(* Logix 5000 AddOnInstructionDefinition export Banner_Q90R2_KD_Param_v4; software revision 33.00; part 3 of 3 *)
(* tags used below, declared in another part *)
   Q90R2KD : Banner_Q90R2KD_v4;
   Port_Data : Banner_IOL_Port_v4;
   Port : DINT;
   Local_Control : DINT;
   Command_Being_Processed : BOOL;
   Index_Write_Inprocess : DINT;
   Inprocess_Index : DINT;
(* Banner_Q90R2_KD_Param_v4, continued *)

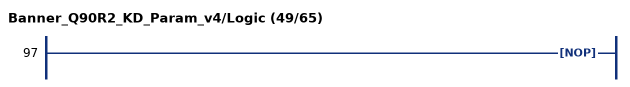
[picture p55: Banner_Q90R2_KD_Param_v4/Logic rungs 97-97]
   97: NOP();
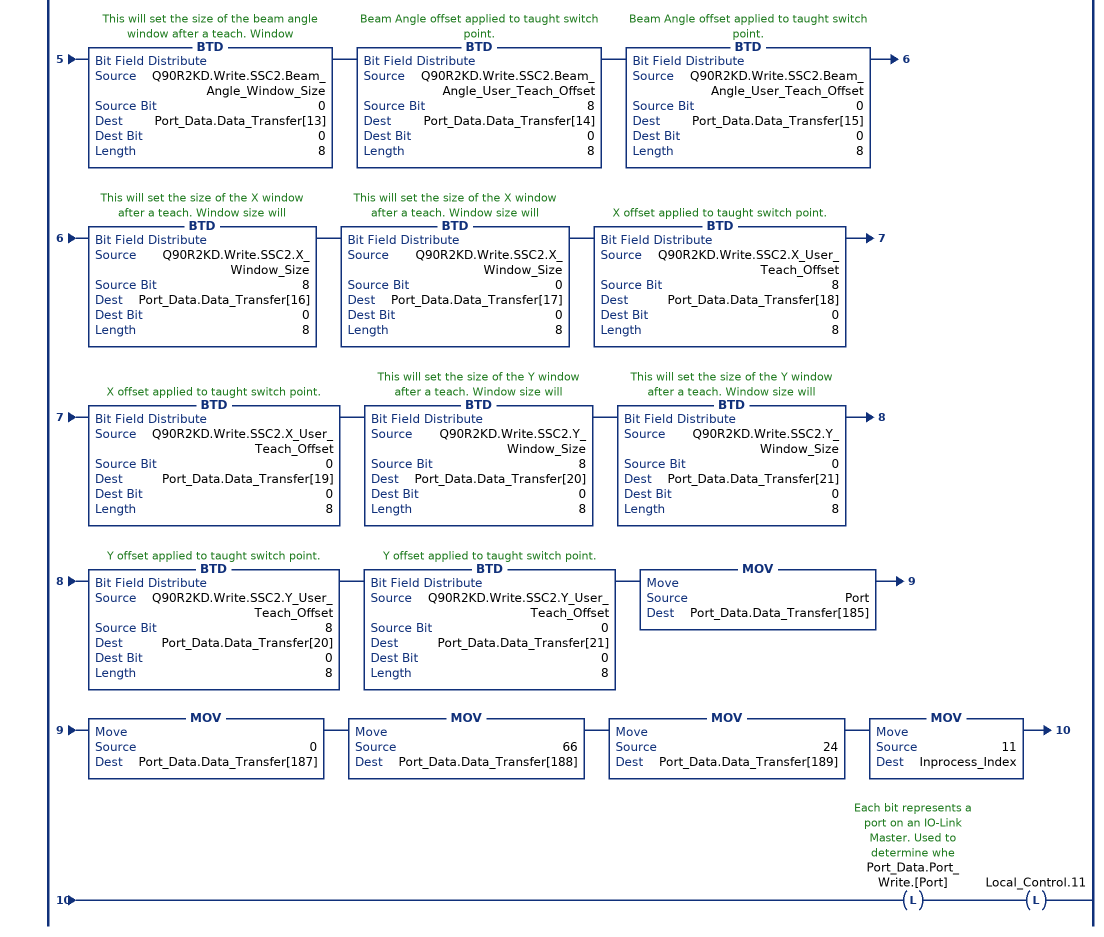
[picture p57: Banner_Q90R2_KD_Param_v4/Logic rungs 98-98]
   // ************************************************************************************************************
   // Section of AOI that controls writing of the SSC2 Vendor Specific Configuration parameter (index 66).
   // ************************************************************************************************************
   98: XIC(Q90R2KD.Initial_Global_Read)XIO(Command_Being_Processed)XIO(Local_Control.11)EQU(Q90R2KD.Command,50)OTL(Command_Being_Processed)BTD(Q90R2KD.Write.SSC2.Delay_On,24,Port_Data.Data_Transfer[0],0,8)BTD(Q90R2KD.Write.SSC2.Delay_On,16,Port_Data.Data_Transfer[1],0,8)BTD(Q90R2KD.Write.SSC2.Delay_On,8,Port_Data.Data_Transfer[2],0,8)BTD(Q90R2KD.Write.SSC2.Delay_On,0,Port_Data.Data_Transfer[3],0,8)BTD(Q90R2KD.Write.SSC2.Delay_Off,24,Port_Data.Data_Transfer[4],0,8)BTD(Q90R2KD.Write.SSC2.Delay_Off,16,Port_Data.Data_Transfer[5],0,8)BTD(Q90R2KD.Write.SSC2.Delay_Off,8,Port_Data.Data_Transfer[6],0,8)BTD(Q90R2KD.Write.SSC2.Delay_Off,0,Port_Data.Data_Transfer[7],0,8)BTD(Q90R2KD.Write.SSC2.Distance_Window_Size,8,Port_Data.Data_Transfer[8],0,8)BTD(Q90R2KD.Write.SSC2.Distance_Window_Size,0,Port_Data.Data_Transfer[9],0,8)BTD(Q90R2KD.Write.SSC2.Distance_User_Teach_Offset,8,Port_Data.Data_Transfer[10],0,8)BTD(Q90R2KD.Write.SSC2.Distance_User_Teach_Offset,0,Port_Data.Data_Transfer[11],0,8)BTD(Q90R2KD.Write.SSC2.Beam_Angle_Window_Size,8,Port_Data.Data_Transfer[12],0,8)BTD(Q90R2KD.Write.SSC2.Beam_Angle_Window_Size,0,Port_Data.Data_Transfer[13],0,8)BTD(Q90R2KD.Write.SSC2.Beam_Angle_User_Teach_Offset,8,Port_Data.Data_Transfer[14],0,8)BTD(Q90R2KD.Write.SSC2.Beam_Angle_User_Teach_Offset,0,Port_Data.Data_Transfer[15],0,8)BTD(Q90R2KD.Write.SSC2.X_Window_Size,8,Port_Data.Data_Transfer[16],0,8)BTD(Q90R2KD.Write.SSC2.X_Window_Size,0,Port_Data.Data_Transfer[17],0,8)BTD(Q90R2KD.Write.SSC2.X_User_Teach_Offset,8,Port_Data.Data_Transfer[18],0,8)BTD(Q90R2KD.Write.SSC2.X_User_Teach_Offset,0,Port_Data.Data_Transfer[19],0,8)BTD(Q90R2KD.Write.SSC2.Y_Window_Size,8,Port_Data.Data_Transfer[20],0,8)BTD(Q90R2KD.Write.SSC2.Y_Window_Size,0,Port_Data.Data_Transfer[21],0,8)BTD(Q90R2KD.Write.SSC2.Y_User_Teach_Offset,8,Port_Data.Data_Transfer[20],0,8)BTD(Q90R2KD.Write.SSC2.Y_User_Teach_Offset,0,Port_Data.Data_Transfer[21],0,8)MOV(Port,Port_Data.Data_Transfer[185])MOV(0,Port_Data.Data_Transfer[187])MOV(66,Port_Data.Data_Transfer[188])MOV(24,Port_Data.Data_Transfer[189])MOV(11,Inprocess_Index)OTL(Port_Data.Port_Write.[Port])OTL(Local_Control.11);
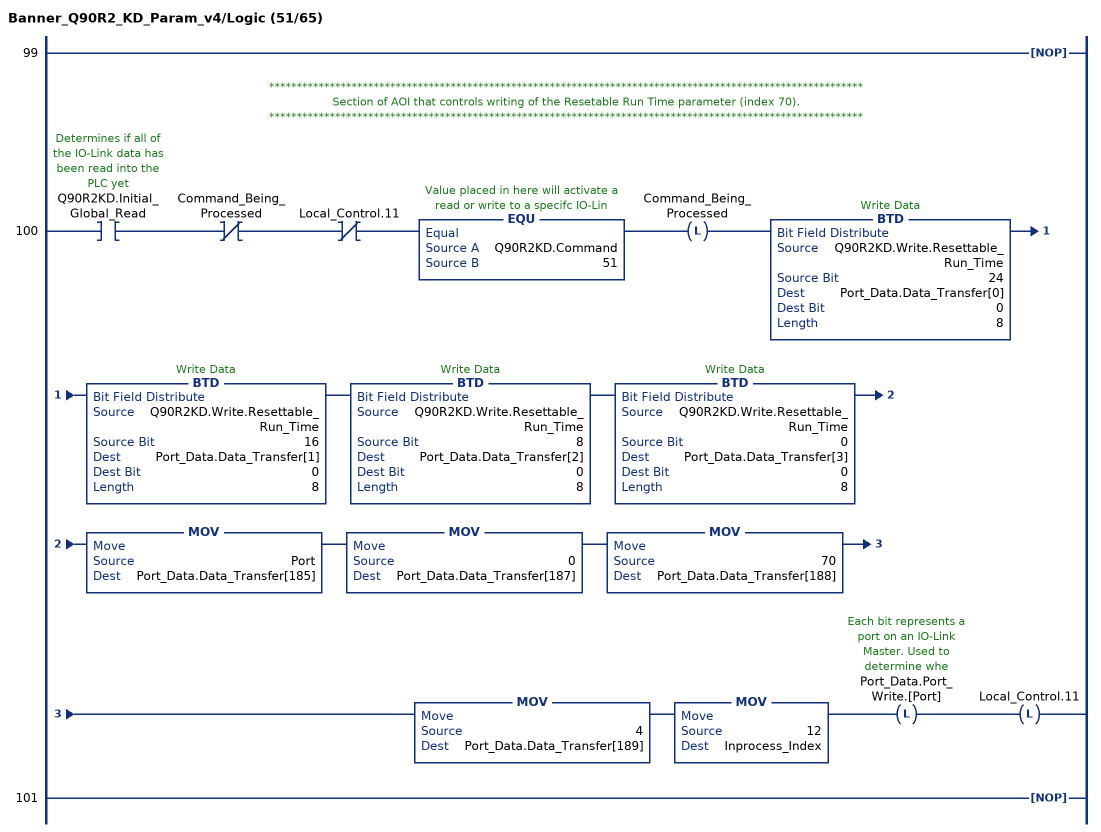
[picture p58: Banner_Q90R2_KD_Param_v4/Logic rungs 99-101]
   99: NOP();
   // ************************************************************************************************************
   // Section of AOI that controls writing of the Resetable Run Time parameter (index 70).
   // ************************************************************************************************************
   100: XIC(Q90R2KD.Initial_Global_Read)XIO(Command_Being_Processed)XIO(Local_Control.11)EQU(Q90R2KD.Command,51)OTL(Command_Being_Processed)BTD(Q90R2KD.Write.Resettable_Run_Time,24,Port_Data.Data_Transfer[0],0,8)BTD(Q90R2KD.Write.Resettable_Run_Time,16,Port_Data.Data_Transfer[1],0,8)BTD(Q90R2KD.Write.Resettable_Run_Time,8,Port_Data.Data_Transfer[2],0,8)BTD(Q90R2KD.Write.Resettable_Run_Time,0,Port_Data.Data_Transfer[3],0,8)MOV(Port,Port_Data.Data_Transfer[185])MOV(0,Port_Data.Data_Transfer[187])MOV(70,Port_Data.Data_Transfer[188])MOV(4,Port_Data.Data_Transfer[189])MOV(12,Inprocess_Index)OTL(Port_Data.Port_Write.[Port])OTL(Local_Control.11);
   101: NOP();
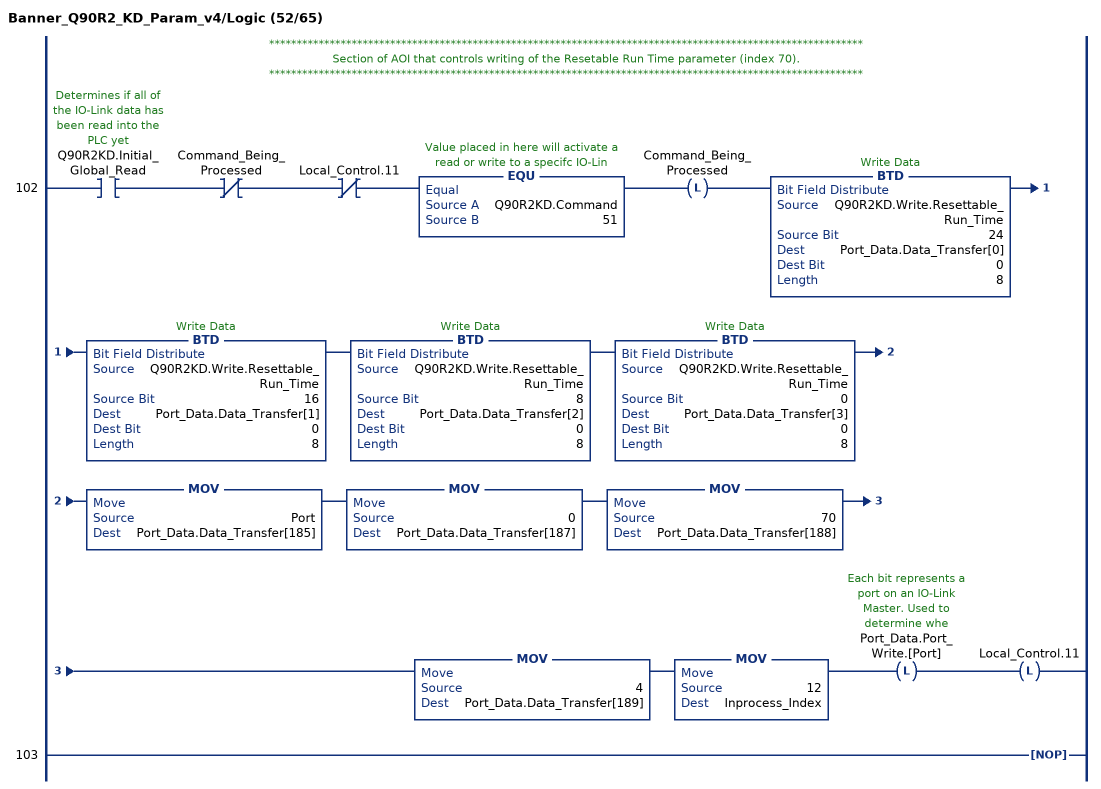
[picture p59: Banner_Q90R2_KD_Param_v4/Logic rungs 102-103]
   // ************************************************************************************************************
   // Section of AOI that controls writing of the Resetable Run Time parameter (index 70).
   // ************************************************************************************************************
   102: XIC(Q90R2KD.Initial_Global_Read)XIO(Command_Being_Processed)XIO(Local_Control.11)EQU(Q90R2KD.Command,51)OTL(Command_Being_Processed)BTD(Q90R2KD.Write.Resettable_Run_Time,24,Port_Data.Data_Transfer[0],0,8)BTD(Q90R2KD.Write.Resettable_Run_Time,16,Port_Data.Data_Transfer[1],0,8)BTD(Q90R2KD.Write.Resettable_Run_Time,8,Port_Data.Data_Transfer[2],0,8)BTD(Q90R2KD.Write.Resettable_Run_Time,0,Port_Data.Data_Transfer[3],0,8)MOV(Port,Port_Data.Data_Transfer[185])MOV(0,Port_Data.Data_Transfer[187])MOV(70,Port_Data.Data_Transfer[188])MOV(4,Port_Data.Data_Transfer[189])MOV(12,Inprocess_Index)OTL(Port_Data.Port_Write.[Port])OTL(Local_Control.11);
   103: NOP();
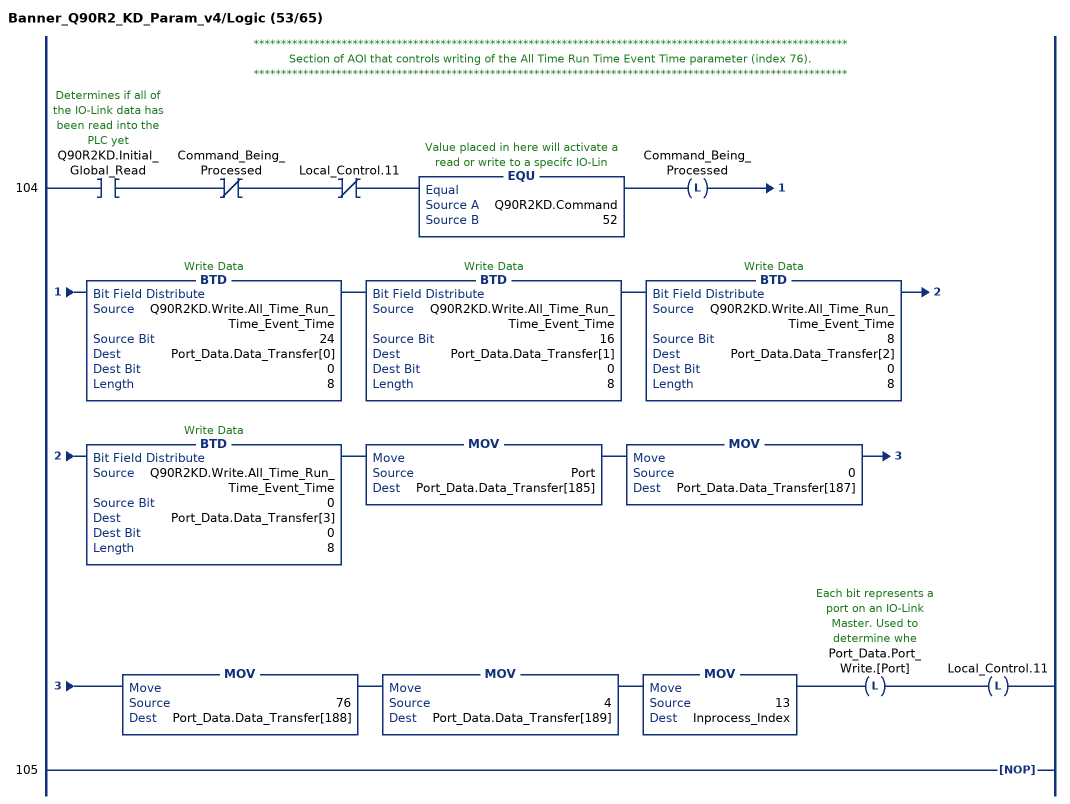
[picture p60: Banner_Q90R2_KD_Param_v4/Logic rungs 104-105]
   // ************************************************************************************************************
   // Section of AOI that controls writing of the All Time Run Time Event Time parameter (index 76).
   // ************************************************************************************************************
   104: XIC(Q90R2KD.Initial_Global_Read)XIO(Command_Being_Processed)XIO(Local_Control.11)EQU(Q90R2KD.Command,52)OTL(Command_Being_Processed)BTD(Q90R2KD.Write.All_Time_Run_Time_Event_Time,24,Port_Data.Data_Transfer[0],0,8)BTD(Q90R2KD.Write.All_Time_Run_Time_Event_Time,16,Port_Data.Data_Transfer[1],0,8)BTD(Q90R2KD.Write.All_Time_Run_Time_Event_Time,8,Port_Data.Data_Transfer[2],0,8)BTD(Q90R2KD.Write.All_Time_Run_Time_Event_Time,0,Port_Data.Data_Transfer[3],0,8)MOV(Port,Port_Data.Data_Transfer[185])MOV(0,Port_Data.Data_Transfer[187])MOV(76,Port_Data.Data_Transfer[188])MOV(4,Port_Data.Data_Transfer[189])MOV(13,Inprocess_Index)OTL(Port_Data.Port_Write.[Port])OTL(Local_Control.11);
   105: NOP();
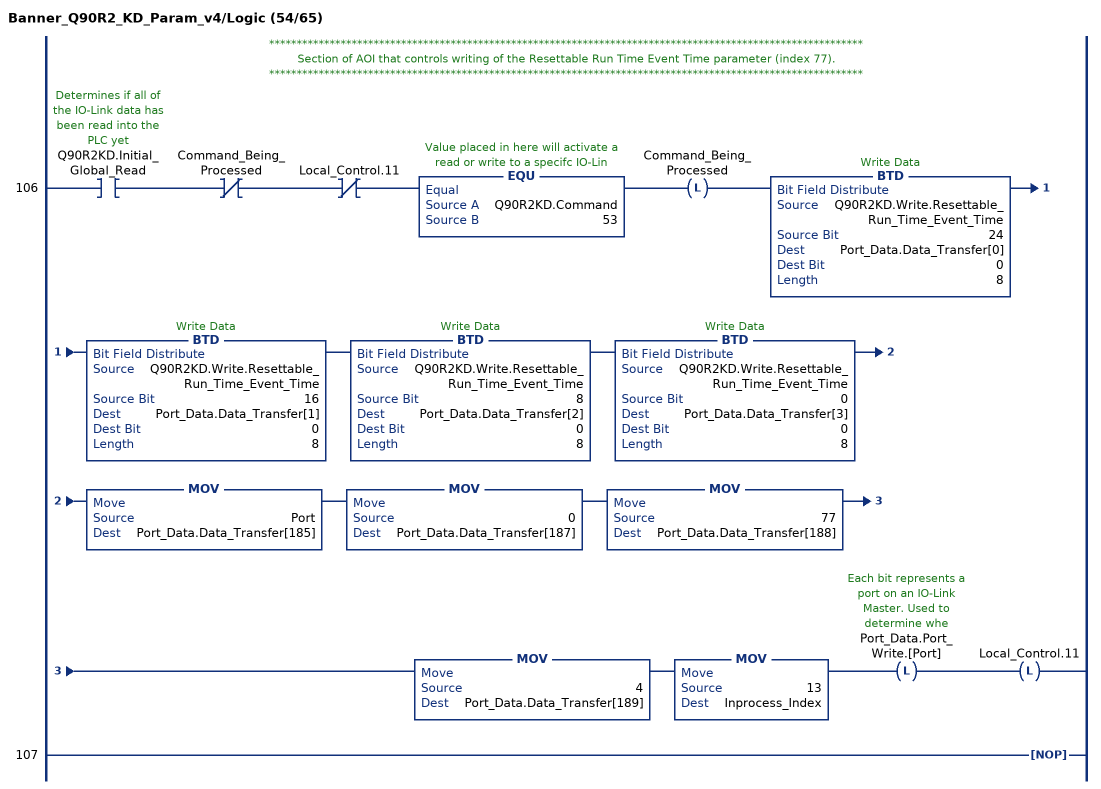
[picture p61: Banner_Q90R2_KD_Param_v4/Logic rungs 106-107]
   // ************************************************************************************************************
   // Section of AOI that controls writing of the Resettable Run Time Event Time parameter (index 77).
   // ************************************************************************************************************
   106: XIC(Q90R2KD.Initial_Global_Read)XIO(Command_Being_Processed)XIO(Local_Control.11)EQU(Q90R2KD.Command,53)OTL(Command_Being_Processed)BTD(Q90R2KD.Write.Resettable_Run_Time_Event_Time,24,Port_Data.Data_Transfer[0],0,8)BTD(Q90R2KD.Write.Resettable_Run_Time_Event_Time,16,Port_Data.Data_Transfer[1],0,8)BTD(Q90R2KD.Write.Resettable_Run_Time_Event_Time,8,Port_Data.Data_Transfer[2],0,8)BTD(Q90R2KD.Write.Resettable_Run_Time_Event_Time,0,Port_Data.Data_Transfer[3],0,8)MOV(Port,Port_Data.Data_Transfer[185])MOV(0,Port_Data.Data_Transfer[187])MOV(77,Port_Data.Data_Transfer[188])MOV(4,Port_Data.Data_Transfer[189])MOV(13,Inprocess_Index)OTL(Port_Data.Port_Write.[Port])OTL(Local_Control.11);
   107: NOP();
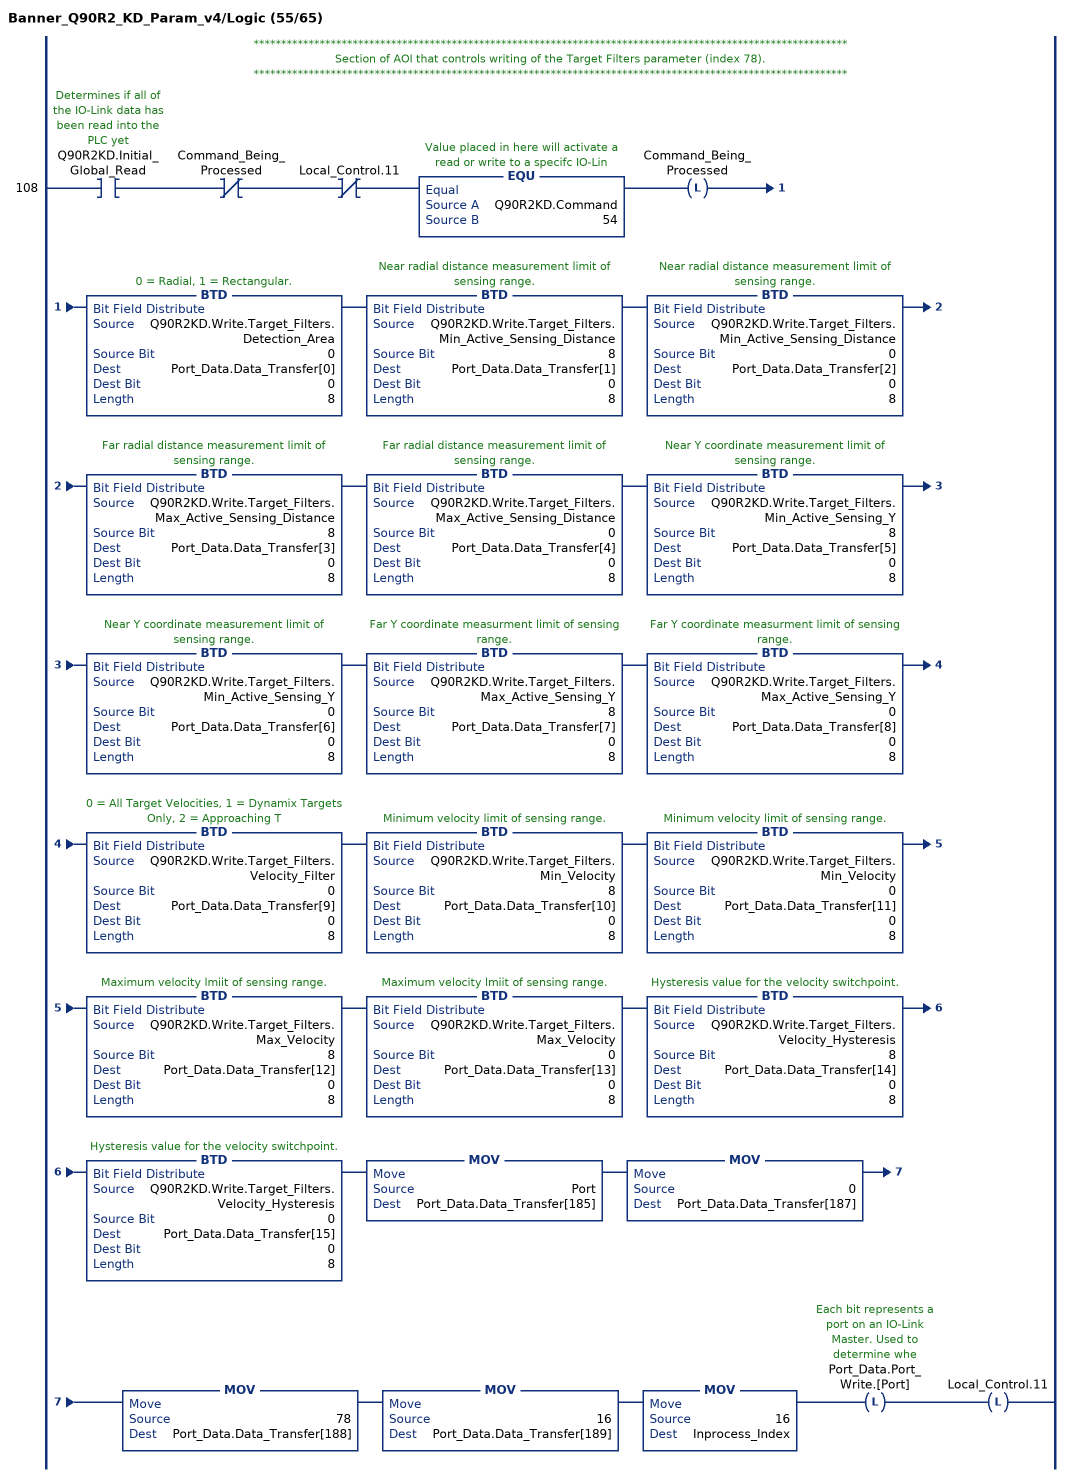
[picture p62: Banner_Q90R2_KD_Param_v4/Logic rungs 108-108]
   // ************************************************************************************************************
   // Section of AOI that controls writing of the Target Filters parameter (index 78).
   // ************************************************************************************************************
   108: XIC(Q90R2KD.Initial_Global_Read)XIO(Command_Being_Processed)XIO(Local_Control.11)EQU(Q90R2KD.Command,54)OTL(Command_Being_Processed)BTD(Q90R2KD.Write.Target_Filters.Detection_Area,0,Port_Data.Data_Transfer[0],0,8)BTD(Q90R2KD.Write.Target_Filters.Min_Active_Sensing_Distance,8,Port_Data.Data_Transfer[1],0,8)BTD(Q90R2KD.Write.Target_Filters.Min_Active_Sensing_Distance,0,Port_Data.Data_Transfer[2],0,8)BTD(Q90R2KD.Write.Target_Filters.Max_Active_Sensing_Distance,8,Port_Data.Data_Transfer[3],0,8)BTD(Q90R2KD.Write.Target_Filters.Max_Active_Sensing_Distance,0,Port_Data.Data_Transfer[4],0,8)BTD(Q90R2KD.Write.Target_Filters.Min_Active_Sensing_Y,8,Port_Data.Data_Transfer[5],0,8)BTD(Q90R2KD.Write.Target_Filters.Min_Active_Sensing_Y,0,Port_Data.Data_Transfer[6],0,8)BTD(Q90R2KD.Write.Target_Filters.Max_Active_Sensing_Y,8,Port_Data.Data_Transfer[7],0,8)BTD(Q90R2KD.Write.Target_Filters.Max_Active_Sensing_Y,0,Port_Data.Data_Transfer[8],0,8)BTD(Q90R2KD.Write.Target_Filters.Velocity_Filter,0,Port_Data.Data_Transfer[9],0,8)BTD(Q90R2KD.Write.Target_Filters.Min_Velocity,8,Port_Data.Data_Transfer[10],0,8)BTD(Q90R2KD.Write.Target_Filters.Min_Velocity,0,Port_Data.Data_Transfer[11],0,8)BTD(Q90R2KD.Write.Target_Filters.Max_Velocity,8,Port_Data.Data_Transfer[12],0,8)BTD(Q90R2KD.Write.Target_Filters.Max_Velocity,0,Port_Data.Data_Transfer[13],0,8)BTD(Q90R2KD.Write.Target_Filters.Velocity_Hysteresis,8,Port_Data.Data_Transfer[14],0,8)BTD(Q90R2KD.Write.Target_Filters.Velocity_Hysteresis,0,Port_Data.Data_Transfer[15],0,8)MOV(Port,Port_Data.Data_Transfer[185])MOV(0,Port_Data.Data_Transfer[187])MOV(78,Port_Data.Data_Transfer[188])MOV(16,Port_Data.Data_Transfer[189])MOV(16,Inprocess_Index)OTL(Port_Data.Port_Write.[Port])OTL(Local_Control.11);
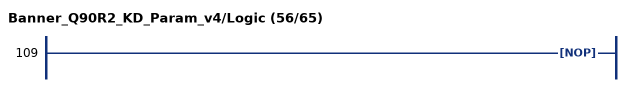
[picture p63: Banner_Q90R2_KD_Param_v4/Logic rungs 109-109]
   109: NOP();
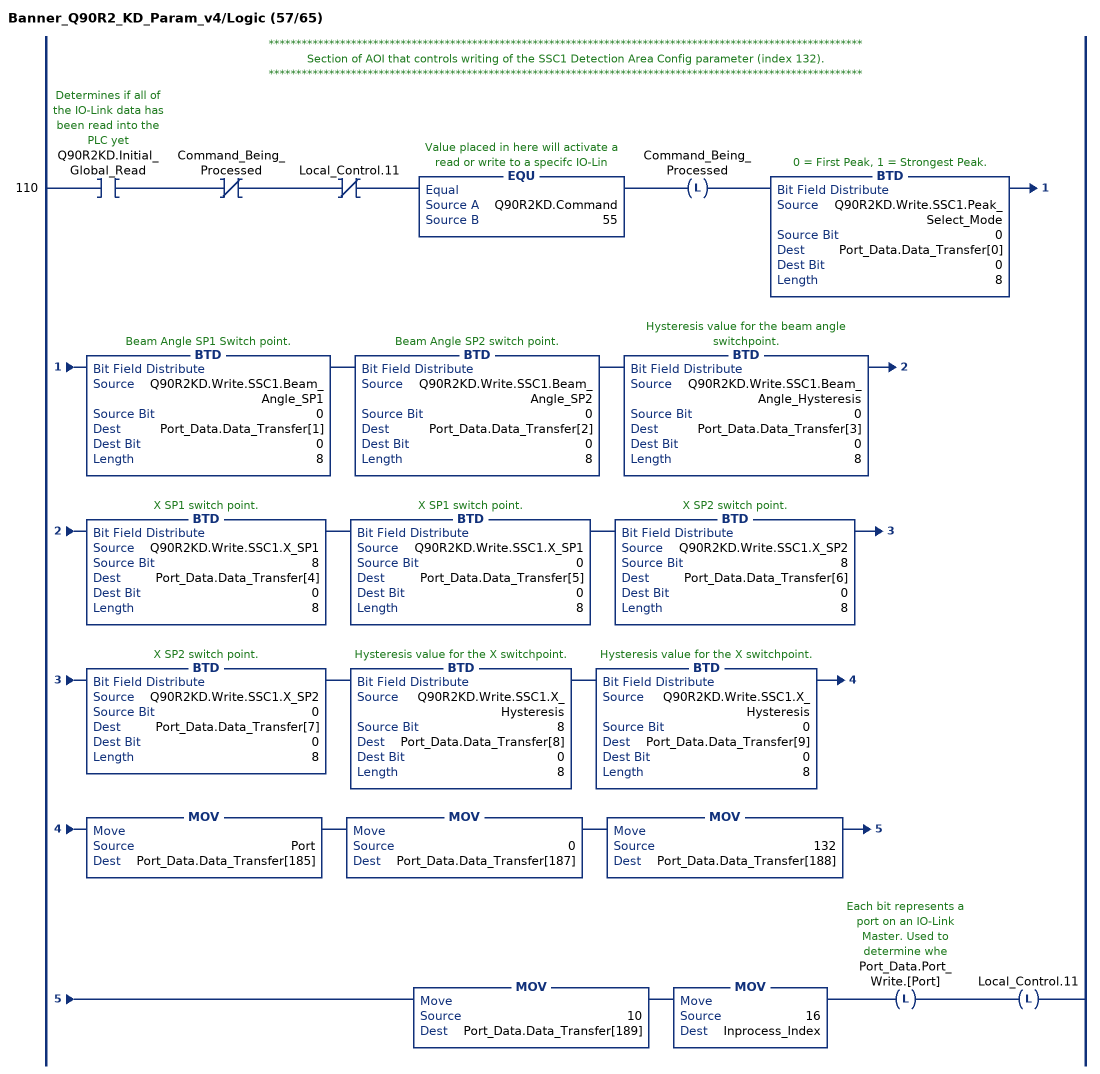
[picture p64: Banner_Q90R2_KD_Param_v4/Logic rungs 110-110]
   // ************************************************************************************************************
   // Section of AOI that controls writing of the SSC1 Detection Area Config parameter (index 132).
   // ************************************************************************************************************
   110: XIC(Q90R2KD.Initial_Global_Read)XIO(Command_Being_Processed)XIO(Local_Control.11)EQU(Q90R2KD.Command,55)OTL(Command_Being_Processed)BTD(Q90R2KD.Write.SSC1.Peak_Select_Mode,0,Port_Data.Data_Transfer[0],0,8)BTD(Q90R2KD.Write.SSC1.Beam_Angle_SP1,0,Port_Data.Data_Transfer[1],0,8)BTD(Q90R2KD.Write.SSC1.Beam_Angle_SP2,0,Port_Data.Data_Transfer[2],0,8)BTD(Q90R2KD.Write.SSC1.Beam_Angle_Hysteresis,0,Port_Data.Data_Transfer[3],0,8)BTD(Q90R2KD.Write.SSC1.X_SP1,8,Port_Data.Data_Transfer[4],0,8)BTD(Q90R2KD.Write.SSC1.X_SP1,0,Port_Data.Data_Transfer[5],0,8)BTD(Q90R2KD.Write.SSC1.X_SP2,8,Port_Data.Data_Transfer[6],0,8)BTD(Q90R2KD.Write.SSC1.X_SP2,0,Port_Data.Data_Transfer[7],0,8)BTD(Q90R2KD.Write.SSC1.X_Hysteresis,8,Port_Data.Data_Transfer[8],0,8)BTD(Q90R2KD.Write.SSC1.X_Hysteresis,0,Port_Data.Data_Transfer[9],0,8)MOV(Port,Port_Data.Data_Transfer[185])MOV(0,Port_Data.Data_Transfer[187])MOV(132,Port_Data.Data_Transfer[188])MOV(10,Port_Data.Data_Transfer[189])MOV(16,Inprocess_Index)OTL(Port_Data.Port_Write.[Port])OTL(Local_Control.11);
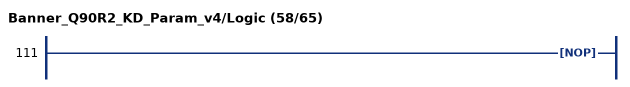
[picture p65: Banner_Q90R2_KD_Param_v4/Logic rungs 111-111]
   111: NOP();
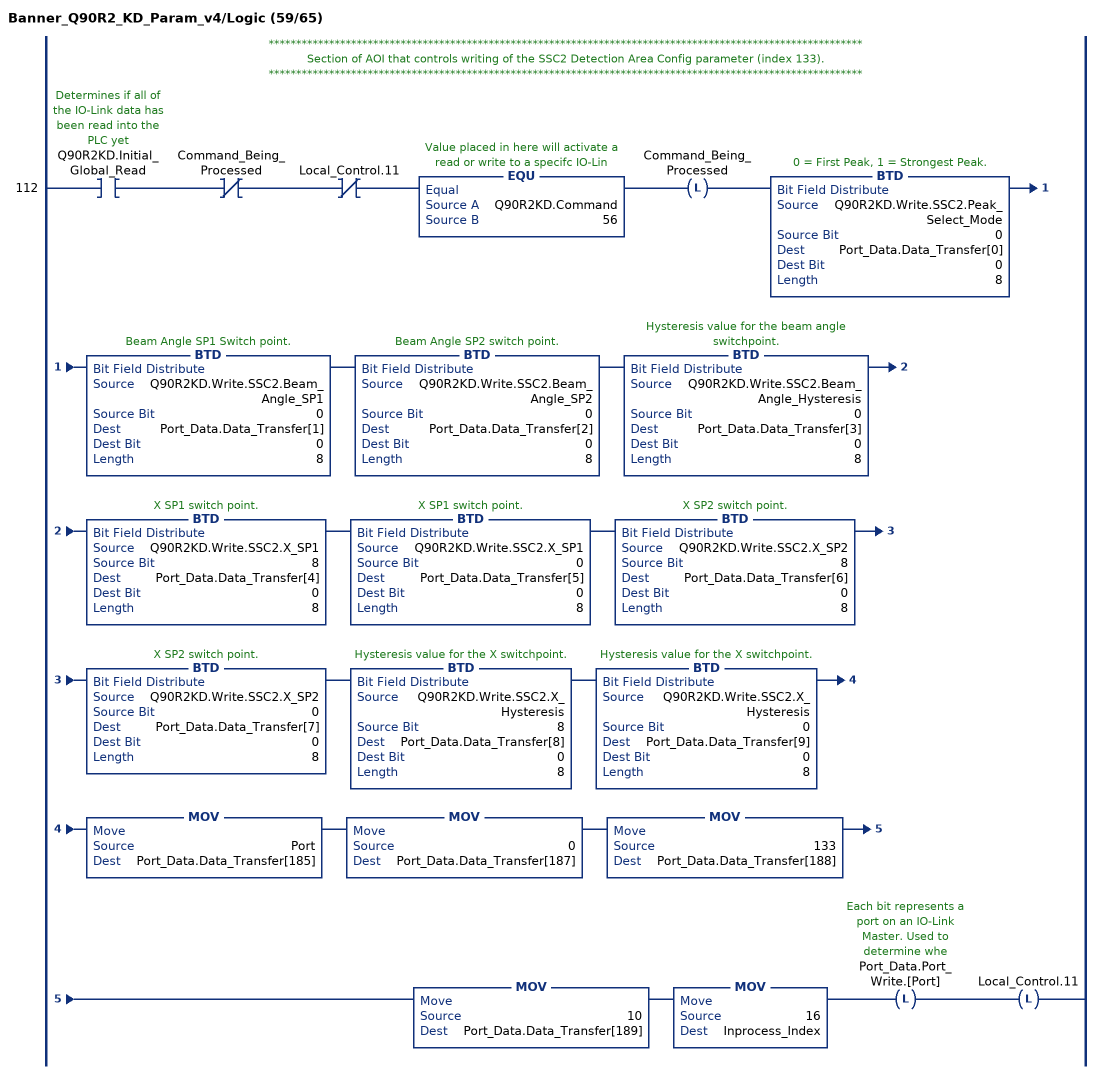
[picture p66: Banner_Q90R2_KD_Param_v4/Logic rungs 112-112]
   // ************************************************************************************************************
   // Section of AOI that controls writing of the SSC2 Detection Area Config parameter (index 133).
   // ************************************************************************************************************
   112: XIC(Q90R2KD.Initial_Global_Read)XIO(Command_Being_Processed)XIO(Local_Control.11)EQU(Q90R2KD.Command,56)OTL(Command_Being_Processed)BTD(Q90R2KD.Write.SSC2.Peak_Select_Mode,0,Port_Data.Data_Transfer[0],0,8)BTD(Q90R2KD.Write.SSC2.Beam_Angle_SP1,0,Port_Data.Data_Transfer[1],0,8)BTD(Q90R2KD.Write.SSC2.Beam_Angle_SP2,0,Port_Data.Data_Transfer[2],0,8)BTD(Q90R2KD.Write.SSC2.Beam_Angle_Hysteresis,0,Port_Data.Data_Transfer[3],0,8)BTD(Q90R2KD.Write.SSC2.X_SP1,8,Port_Data.Data_Transfer[4],0,8)BTD(Q90R2KD.Write.SSC2.X_SP1,0,Port_Data.Data_Transfer[5],0,8)BTD(Q90R2KD.Write.SSC2.X_SP2,8,Port_Data.Data_Transfer[6],0,8)BTD(Q90R2KD.Write.SSC2.X_SP2,0,Port_Data.Data_Transfer[7],0,8)BTD(Q90R2KD.Write.SSC2.X_Hysteresis,8,Port_Data.Data_Transfer[8],0,8)BTD(Q90R2KD.Write.SSC2.X_Hysteresis,0,Port_Data.Data_Transfer[9],0,8)MOV(Port,Port_Data.Data_Transfer[185])MOV(0,Port_Data.Data_Transfer[187])MOV(133,Port_Data.Data_Transfer[188])MOV(10,Port_Data.Data_Transfer[189])MOV(16,Inprocess_Index)OTL(Port_Data.Port_Write.[Port])OTL(Local_Control.11);
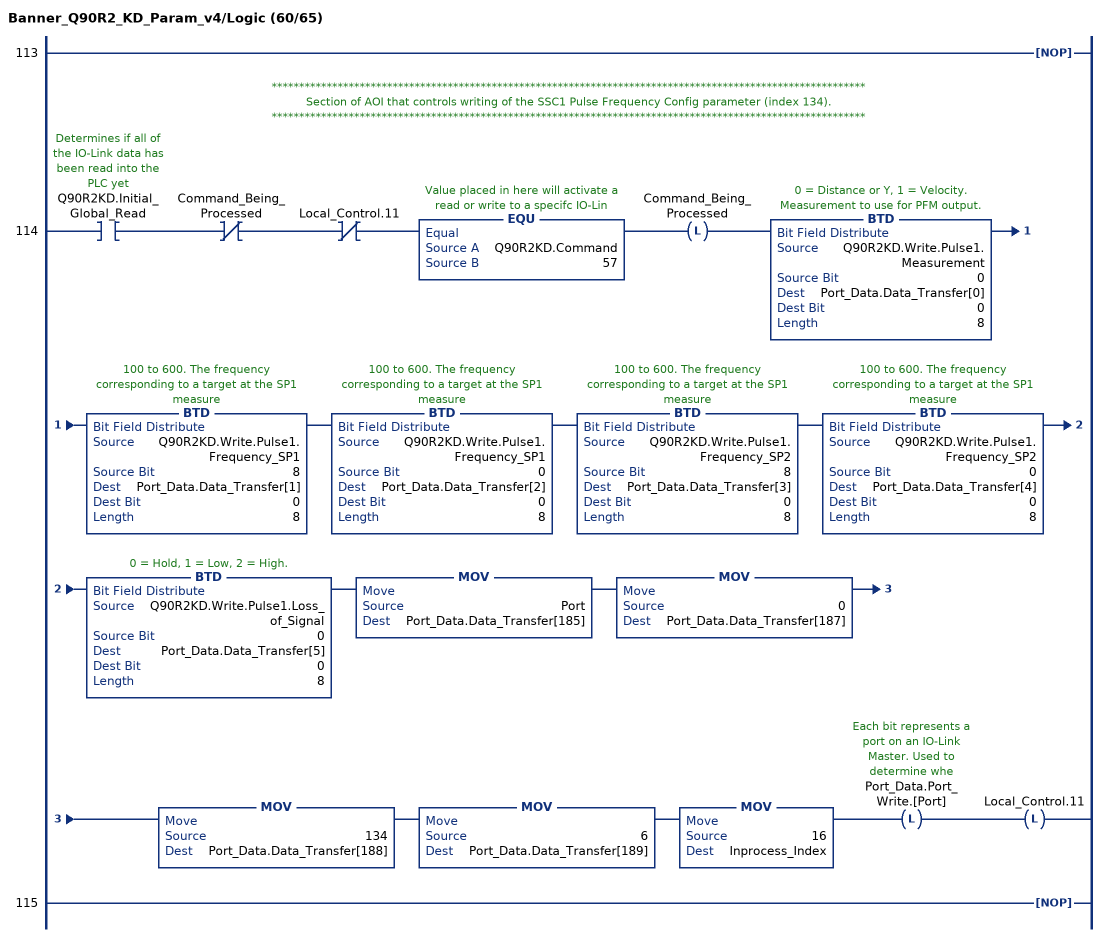
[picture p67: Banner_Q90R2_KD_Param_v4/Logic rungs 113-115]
   113: NOP();
   // ************************************************************************************************************
   // Section of AOI that controls writing of the SSC1 Pulse Frequency Config parameter (index 134).
   // ************************************************************************************************************
   114: XIC(Q90R2KD.Initial_Global_Read)XIO(Command_Being_Processed)XIO(Local_Control.11)EQU(Q90R2KD.Command,57)OTL(Command_Being_Processed)BTD(Q90R2KD.Write.Pulse1.Measurement,0,Port_Data.Data_Transfer[0],0,8)BTD(Q90R2KD.Write.Pulse1.Frequency_SP1,8,Port_Data.Data_Transfer[1],0,8)BTD(Q90R2KD.Write.Pulse1.Frequency_SP1,0,Port_Data.Data_Transfer[2],0,8)BTD(Q90R2KD.Write.Pulse1.Frequency_SP2,8,Port_Data.Data_Transfer[3],0,8)BTD(Q90R2KD.Write.Pulse1.Frequency_SP2,0,Port_Data.Data_Transfer[4],0,8)BTD(Q90R2KD.Write.Pulse1.Loss_of_Signal,0,Port_Data.Data_Transfer[5],0,8)MOV(Port,Port_Data.Data_Transfer[185])MOV(0,Port_Data.Data_Transfer[187])MOV(134,Port_Data.Data_Transfer[188])MOV(6,Port_Data.Data_Transfer[189])MOV(16,Inprocess_Index)OTL(Port_Data.Port_Write.[Port])OTL(Local_Control.11);
   115: NOP();
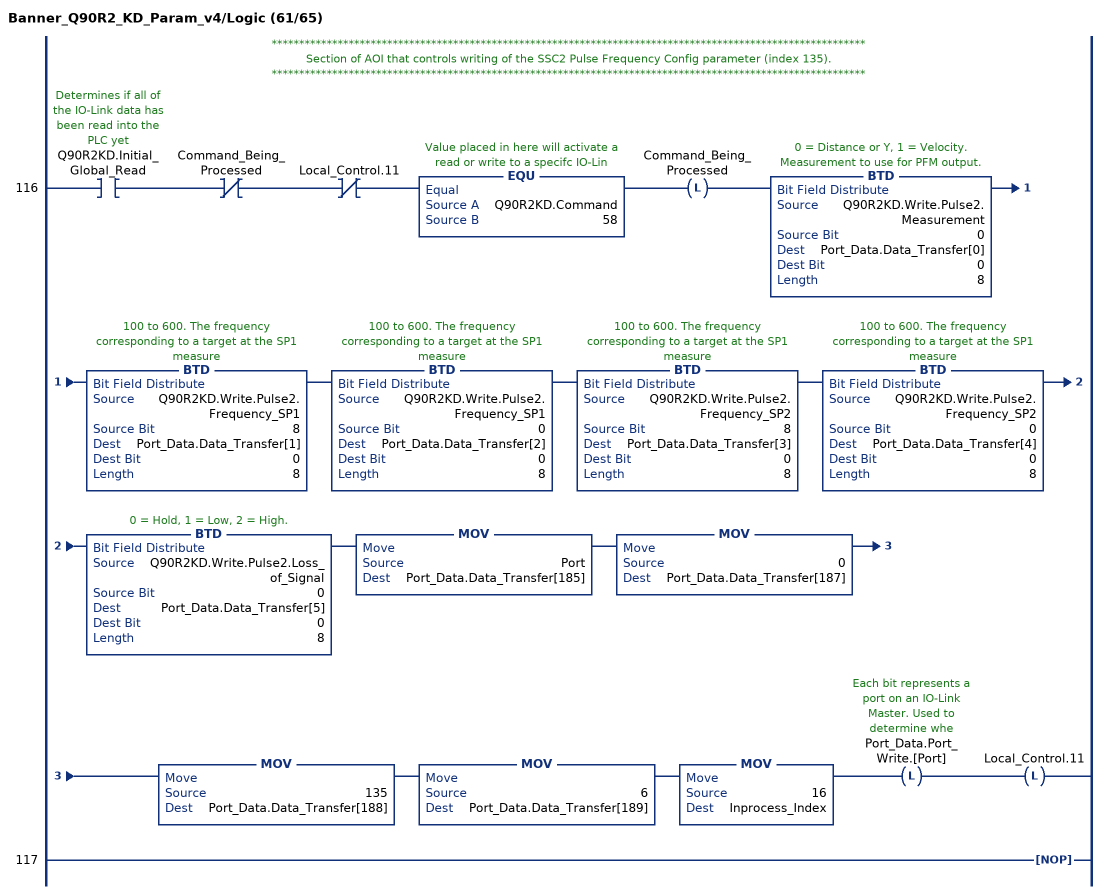
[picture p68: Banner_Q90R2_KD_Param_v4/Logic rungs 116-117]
   // ************************************************************************************************************
   // Section of AOI that controls writing of the SSC2 Pulse Frequency Config parameter (index 135).
   // ************************************************************************************************************
   116: XIC(Q90R2KD.Initial_Global_Read)XIO(Command_Being_Processed)XIO(Local_Control.11)EQU(Q90R2KD.Command,58)OTL(Command_Being_Processed)BTD(Q90R2KD.Write.Pulse2.Measurement,0,Port_Data.Data_Transfer[0],0,8)BTD(Q90R2KD.Write.Pulse2.Frequency_SP1,8,Port_Data.Data_Transfer[1],0,8)BTD(Q90R2KD.Write.Pulse2.Frequency_SP1,0,Port_Data.Data_Transfer[2],0,8)BTD(Q90R2KD.Write.Pulse2.Frequency_SP2,8,Port_Data.Data_Transfer[3],0,8)BTD(Q90R2KD.Write.Pulse2.Frequency_SP2,0,Port_Data.Data_Transfer[4],0,8)BTD(Q90R2KD.Write.Pulse2.Loss_of_Signal,0,Port_Data.Data_Transfer[5],0,8)MOV(Port,Port_Data.Data_Transfer[185])MOV(0,Port_Data.Data_Transfer[187])MOV(135,Port_Data.Data_Transfer[188])MOV(6,Port_Data.Data_Transfer[189])MOV(16,Inprocess_Index)OTL(Port_Data.Port_Write.[Port])OTL(Local_Control.11);
   117: NOP();
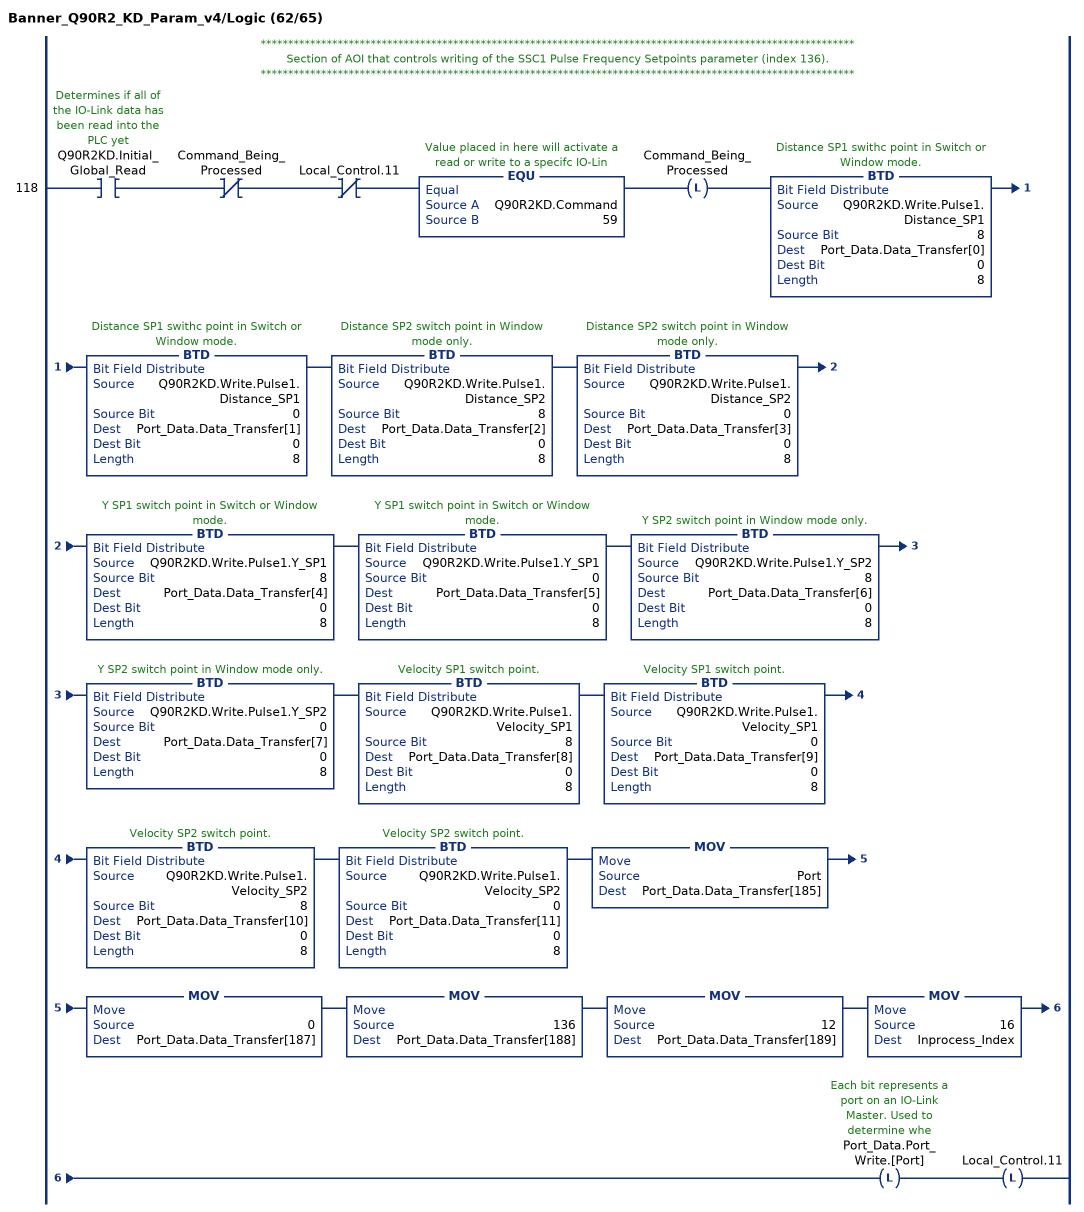
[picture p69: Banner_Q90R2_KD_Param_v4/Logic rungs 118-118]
   // ************************************************************************************************************
   // Section of AOI that controls writing of the SSC1 Pulse Frequency Setpoints parameter (index 136).
   // ************************************************************************************************************
   118: XIC(Q90R2KD.Initial_Global_Read)XIO(Command_Being_Processed)XIO(Local_Control.11)EQU(Q90R2KD.Command,59)OTL(Command_Being_Processed)BTD(Q90R2KD.Write.Pulse1.Distance_SP1,8,Port_Data.Data_Transfer[0],0,8)BTD(Q90R2KD.Write.Pulse1.Distance_SP1,0,Port_Data.Data_Transfer[1],0,8)BTD(Q90R2KD.Write.Pulse1.Distance_SP2,8,Port_Data.Data_Transfer[2],0,8)BTD(Q90R2KD.Write.Pulse1.Distance_SP2,0,Port_Data.Data_Transfer[3],0,8)BTD(Q90R2KD.Write.Pulse1.Y_SP1,8,Port_Data.Data_Transfer[4],0,8)BTD(Q90R2KD.Write.Pulse1.Y_SP1,0,Port_Data.Data_Transfer[5],0,8)BTD(Q90R2KD.Write.Pulse1.Y_SP2,8,Port_Data.Data_Transfer[6],0,8)BTD(Q90R2KD.Write.Pulse1.Y_SP2,0,Port_Data.Data_Transfer[7],0,8)BTD(Q90R2KD.Write.Pulse1.Velocity_SP1,8,Port_Data.Data_Transfer[8],0,8)BTD(Q90R2KD.Write.Pulse1.Velocity_SP1,0,Port_Data.Data_Transfer[9],0,8)BTD(Q90R2KD.Write.Pulse1.Velocity_SP2,8,Port_Data.Data_Transfer[10],0,8)BTD(Q90R2KD.Write.Pulse1.Velocity_SP2,0,Port_Data.Data_Transfer[11],0,8)MOV(Port,Port_Data.Data_Transfer[185])MOV(0,Port_Data.Data_Transfer[187])MOV(136,Port_Data.Data_Transfer[188])MOV(12,Port_Data.Data_Transfer[189])MOV(16,Inprocess_Index)OTL(Port_Data.Port_Write.[Port])OTL(Local_Control.11);
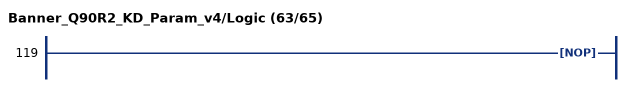
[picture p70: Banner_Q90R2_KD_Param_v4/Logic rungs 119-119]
   119: NOP();
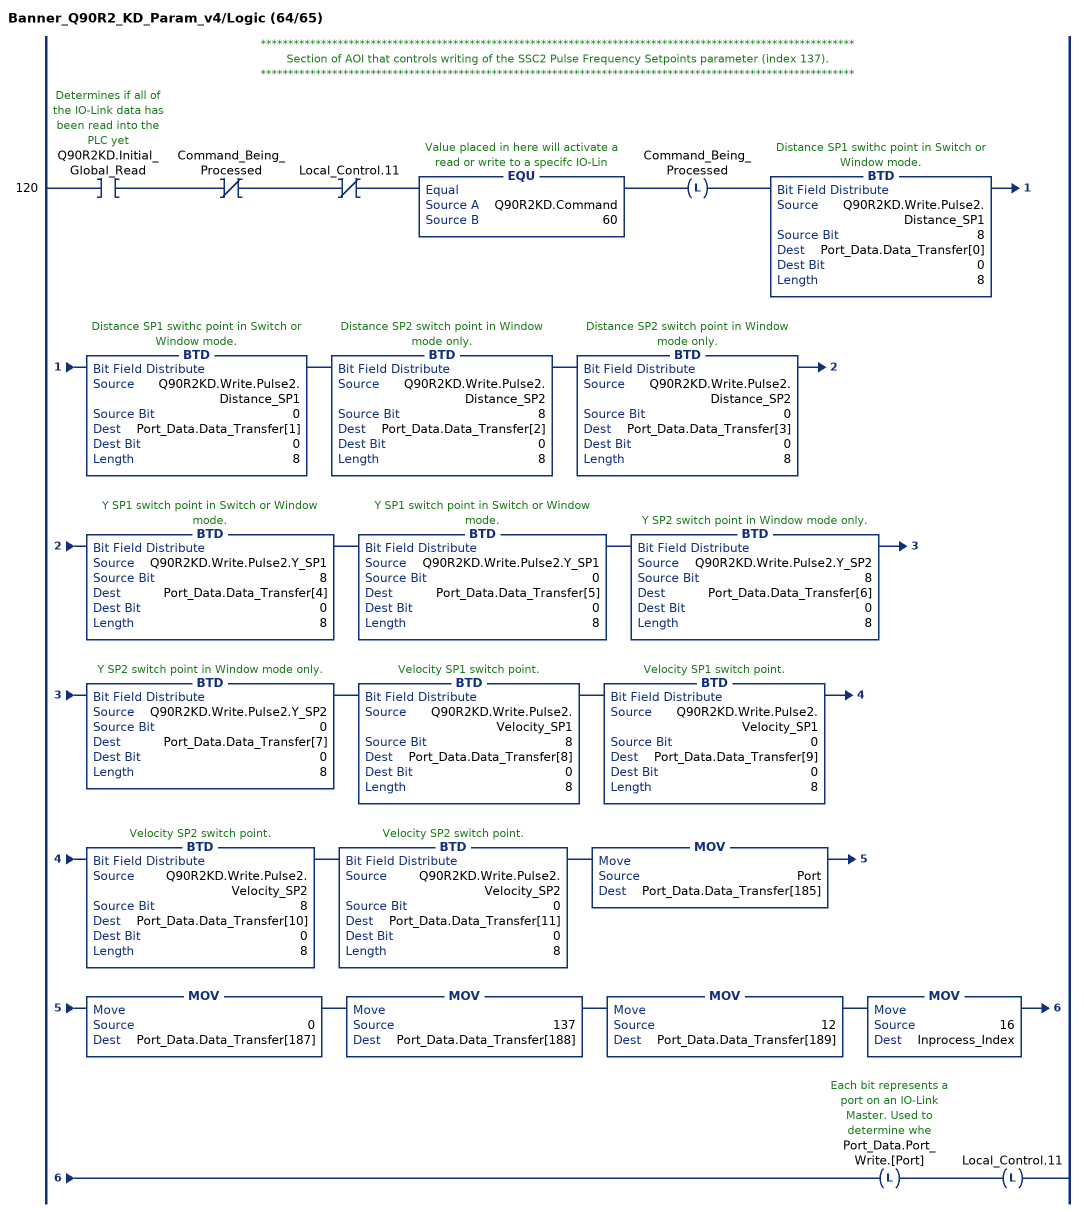
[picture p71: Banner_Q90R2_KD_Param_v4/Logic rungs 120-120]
   // ************************************************************************************************************
   // Section of AOI that controls writing of the SSC2 Pulse Frequency Setpoints parameter (index 137).
   // ************************************************************************************************************
   120: XIC(Q90R2KD.Initial_Global_Read)XIO(Command_Being_Processed)XIO(Local_Control.11)EQU(Q90R2KD.Command,60)OTL(Command_Being_Processed)BTD(Q90R2KD.Write.Pulse2.Distance_SP1,8,Port_Data.Data_Transfer[0],0,8)BTD(Q90R2KD.Write.Pulse2.Distance_SP1,0,Port_Data.Data_Transfer[1],0,8)BTD(Q90R2KD.Write.Pulse2.Distance_SP2,8,Port_Data.Data_Transfer[2],0,8)BTD(Q90R2KD.Write.Pulse2.Distance_SP2,0,Port_Data.Data_Transfer[3],0,8)BTD(Q90R2KD.Write.Pulse2.Y_SP1,8,Port_Data.Data_Transfer[4],0,8)BTD(Q90R2KD.Write.Pulse2.Y_SP1,0,Port_Data.Data_Transfer[5],0,8)BTD(Q90R2KD.Write.Pulse2.Y_SP2,8,Port_Data.Data_Transfer[6],0,8)BTD(Q90R2KD.Write.Pulse2.Y_SP2,0,Port_Data.Data_Transfer[7],0,8)BTD(Q90R2KD.Write.Pulse2.Velocity_SP1,8,Port_Data.Data_Transfer[8],0,8)BTD(Q90R2KD.Write.Pulse2.Velocity_SP1,0,Port_Data.Data_Transfer[9],0,8)BTD(Q90R2KD.Write.Pulse2.Velocity_SP2,8,Port_Data.Data_Transfer[10],0,8)BTD(Q90R2KD.Write.Pulse2.Velocity_SP2,0,Port_Data.Data_Transfer[11],0,8)MOV(Port,Port_Data.Data_Transfer[185])MOV(0,Port_Data.Data_Transfer[187])MOV(137,Port_Data.Data_Transfer[188])MOV(12,Port_Data.Data_Transfer[189])MOV(16,Inprocess_Index)OTL(Port_Data.Port_Write.[Port])OTL(Local_Control.11);
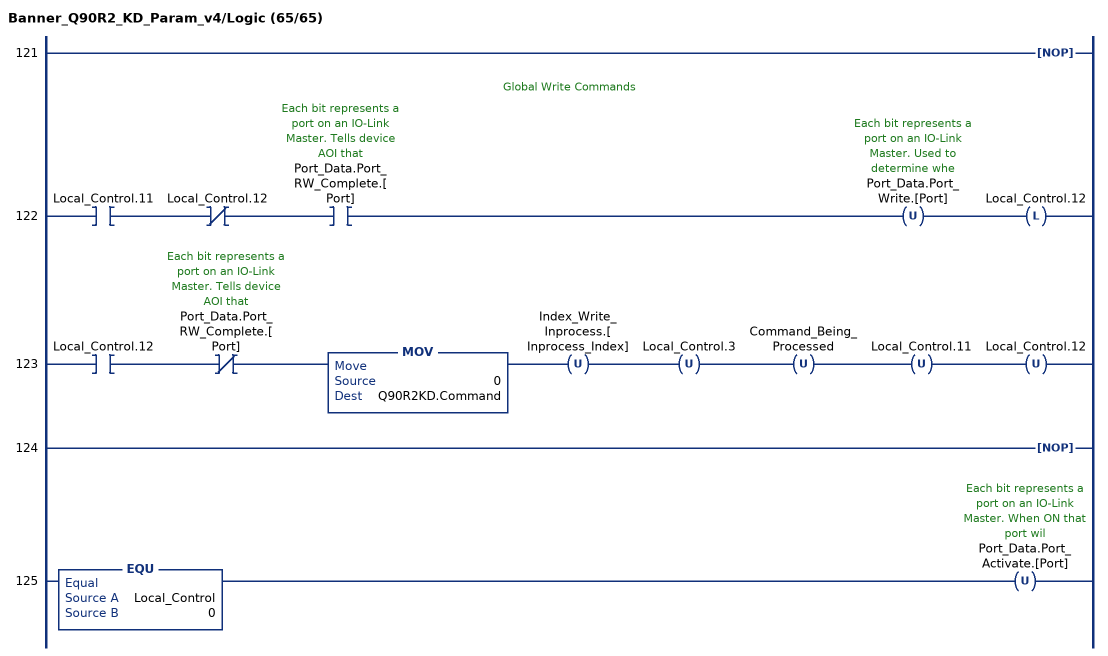
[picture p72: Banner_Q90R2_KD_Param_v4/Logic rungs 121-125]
   121: NOP();
   // Global Write Commands
   122: XIC(Local_Control.11)XIO(Local_Control.12)XIC(Port_Data.Port_RW_Complete.[Port])OTU(Port_Data.Port_Write.[Port])OTL(Local_Control.12);
   123: XIC(Local_Control.12)XIO(Port_Data.Port_RW_Complete.[Port])MOV(0,Q90R2KD.Command)OTU(Index_Write_Inprocess.[Inprocess_Index])OTU(Local_Control.3)OTU(Command_Being_Processed)OTU(Local_Control.11)OTU(Local_Control.12);
   124: NOP();
   125: EQU(Local_Control,0)OTU(Port_Data.Port_Activate.[Port]);
END_ROUTINE
END_ADD_ON_INSTRUCTION
